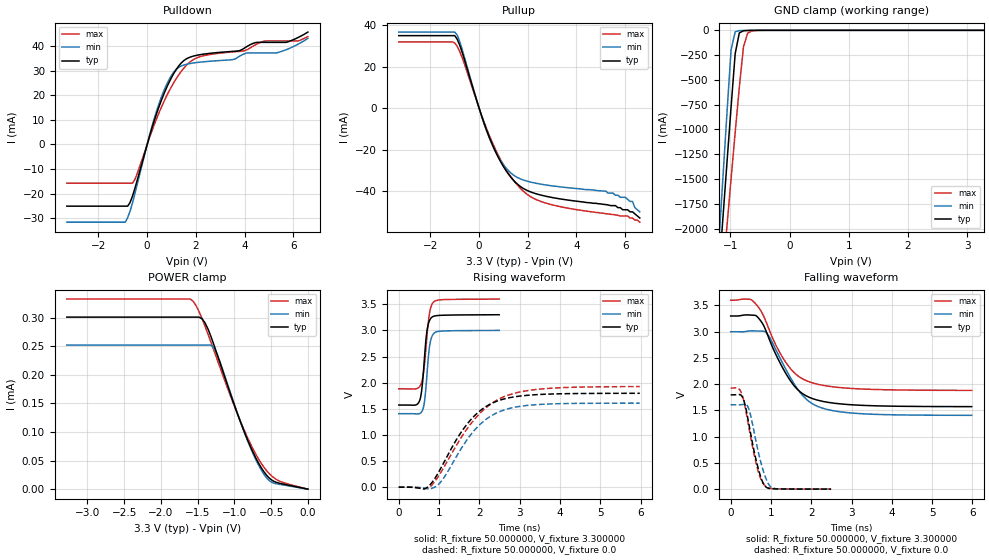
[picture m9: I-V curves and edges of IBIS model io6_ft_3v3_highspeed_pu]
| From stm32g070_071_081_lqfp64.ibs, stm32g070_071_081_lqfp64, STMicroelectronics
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|   Model io6_ft_3v3_highspeed_pu
[Model]  io6_ft_3v3_highspeed_pu
Model_type I/O
Polarity   Non-Inverting
Enable   Active-Low
Vinl =   0.990000V
Vinh =   2.310000V
Vmeas =  1.650000V
Cref =   50.000000pF
Rref =   100.000000M
Vref =   0.0V
C_comp   1.290400pF   1.272500pF   1.305600pF
[Temperature Range]   25.000000   -40.000000   0.125000k
[Pullup Reference]   3.300000V   3.000000V   3.600000V
[Pulldown Reference]   0.0V   0.0V   0.0V
[POWER Clamp Reference]   3.300000V   3.000000V   3.600000V
[GND Clamp Reference]   0.0V   0.0V   0.0V
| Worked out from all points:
|   slope of the pulldown table from 0 to 0.495 V, typ, clamps not added: 31.8 ohm
|   slope of the pullup table from 0 to 0.495 V, typ, clamps not added: 30.4 ohm
|   GND clamp passes 1 mA (typ) near -0.65 V on its own axis
|   rising waveform, R_fixture 50.000000, V_fixture 3.300000: 20-80 % time 115ps typ, 110ps min, 129ps max; typ from 1.57 V to 3.3 V
|   rising waveform, R_fixture 50.000000, V_fixture 0.0: 20-80 % time 937ps typ, 912ps min, 1.08ns max; typ from 0.002 V to 1.8 V
|   falling waveform, R_fixture 50.000000, V_fixture 3.300000: 20-80 % time 727ps typ, 757ps min, 727ps max; typ from 3.3 V to 1.57 V
|   falling waveform, R_fixture 50.000000, V_fixture 0.0: 20-80 % time 293ps typ, 290ps min, 303ps max; typ from 1.8 V to 0.002 V
[Pulldown]
|Voltage   I(typ)   I(min)   I(max)
-3.3V     -25.03mA   -31.54mA   -15.7mA
-900mV    -25.03mA   -31.54mA   -15.7mA
-700mV    -23.48mA   -26.95mA   -15.7mA
-500mV    -17.69mA   -19.75mA   -14.07mA
100mV     3.479mA    3.853mA    2.862mA
500mV     15.71mA    16.96mA    13.17mA
900mV     25.22mA    26.33mA    21.66mA
1.3V      31.91mA    31.32mA    28.29mA
2.2V      36.48mA    33.43mA    35.69mA
4.1V      39.76mA    37.15mA    38.42mA
5.3V      41.43mA    37.15mA    42.02mA
6.6V      45.6mA     43.04mA    43.74mA
[Pullup]
|Voltage   I(typ)   I(min)   I(max)
-3.3V     34.92mA    36.63mA    31.91mA
-1V       34.92mA    36.63mA    31.44mA
-800mV    30.46mA    32.23mA    27.37mA
100mV     -3.672mA   -3.825mA   -3.371mA
500mV     -16.4mA    -16.57mA   -15.42mA
1.1V      -30.05mA   -28.8mA    -29.38mA
1.7V      -37.83mA   -34.15mA   -38.73mA
2.8V      -42.64mA   -37.15mA   -46mA
5.2V      -46.5mA    -40mA      -50.9mA
6.3V      -50mA      -45mA      -53mA
6.4V      -51mA      -48mA      -54mA
6.6V      -53mA      -50mA      -55mA
[GND_clamp]
|Voltage   I(typ)   I(min)   I(max)
-3.3V     -9.61A     -9.635A    -9.699A
-1.2V     -2.493A    -2.184A    -2.958A
-1.13V    -1.917A    -1.512A    -2.469A
-1.06V    -1.345A    -845.6mA   -1.983A
-990mV    -779.8mA   -200.2mA   -1.503A
-920mV    -235.5mA   -14.18mA   -1.03A
-850mV    -26.06mA   -3.338mA   -574.2mA
-780mV    -4.499mA   -1.808mA   -166.4mA
-710mV    -1.722mA   -869.6uA   -29.45mA
-640mV    -806.7uA   -283.7uA   -6.281mA
3.28V     0A         0A         0A
[POWER_clamp]
|Voltage   I(typ)   I(min)   I(max)
-3.28V    300.8uA    252uA      332.4uA
-1.6V     300.8uA    252uA      332.4uA
-1.56V    300.8uA    252uA      328.4uA
-1.44V    297.9uA    252uA      298.3uA
-1.36V    280.4uA    252uA      271.4uA
-1.28V    252.9uA    246.9uA    243.1uA
-1.2V     222.5uA    224.3uA    214.5uA
-920mV    118.6uA    118.8uA    119.5uA
-680mV    47.6uA     44.33uA    54.63uA
-560mV    24.08uA    19.48uA    32.08uA
-480mV    14.89uA    11.29uA    21.67uA
0V        0A         0A         0A
[Ramp]
| variable   typ   min   max
dV/dt_r  1.07552/0.93429n   0.96306/0.90911n   1.14953/1.06800n
dV/dt_f  1.03422/0.72440n   0.95490/0.75402n   1.02804/0.72299n
R_load = 50.000000
[Rising Waveform]
R_fixture= 50.000000
V_fixture= 3.300000
V_fixture_min= 3.000000
V_fixture_max= 3.600000
|time   V(typ)   V(min)   V(max)
0s        1.573V     1.408V     1.883V
445.4ps   1.582V     1.403V     1.887V
555.6ps   1.779V     1.43V      1.977V
590.6ps   2.008V     1.474V     2.077V
630.6ps   2.39V      1.597V     2.296V
695.7ps   2.966V     2.108V     2.848V
750.8ps   3.166V     2.613V     3.264V
810.8ps   3.245V     2.859V     3.474V
1.006ns   3.287V     2.984V     3.583V
2.492ns   3.3V       3V         3.6V
[Rising Waveform]
R_fixture= 50.000000
V_fixture= 0.0
V_fixture_min= 0.0
V_fixture_max= 0.0
|time   V(typ)   V(min)   V(max)
0s        1.677mV    1.094mV    2.442mV
624.6ps   -34.37mV   -13.49mV   -19.67mV
780.8ps   51.26mV    -31.16mV   7.913mV
1.081ns   417.8mV    140.4mV    331.8mV
1.417ns   892.3mV    568.2mV    783.3mV
1.718ns   1.229V     934.1mV    1.143V
2.054ns   1.485V     1.228V     1.443V
2.45ns    1.651V     1.429V     1.672V
3.423ns   1.772V     1.58V      1.872V
5.982ns   1.797V     1.608V     1.926V
[Falling Waveform]
R_fixture= 50.000000
V_fixture= 3.300000
V_fixture_min= 3.000000
V_fixture_max= 3.600000
|time   V(typ)   V(min)   V(max)
0s        3.3V       3V         3.6V
504.5ps   3.317V     3.017V     3.612V
648.6ps   3.295V     3.014V     3.507V
864.9ps   3.04V      2.995V     3.217V
1.369ns   2.205V     2.284V     2.416V
1.646ns   1.911V     1.925V     2.173V
1.898ns   1.77V      1.7V       2.061V
2.33ns    1.667V     1.532V     1.974V
2.943ns   1.611V     1.455V     1.922V
5.982ns   1.573V     1.408V     1.883V
[Falling Waveform]
R_fixture= 50.000000
V_fixture= 0.0
V_fixture_min= 0.0
V_fixture_max= 0.0
|time   V(typ)   V(min)   V(max)
0s        1.797V     1.608V     1.926V
245.2ps   1.797V     1.61V      1.87V
330.3ps   1.682V     1.617V     1.664V
430.4ps   1.332V     1.567V     1.27V
500.5ps   1.041V     1.392V     976.9mV
665.7ps   449.3mV    779.2mV    390.1mV
860.9ps   53.61mV    234.1mV    62.16mV
961ps     14.42mV    73.21mV    20.61mV
1.076ns   7.249mV    16.62mV    8.974mV
2.492ns   1.677mV    1.094mV    2.442mV
